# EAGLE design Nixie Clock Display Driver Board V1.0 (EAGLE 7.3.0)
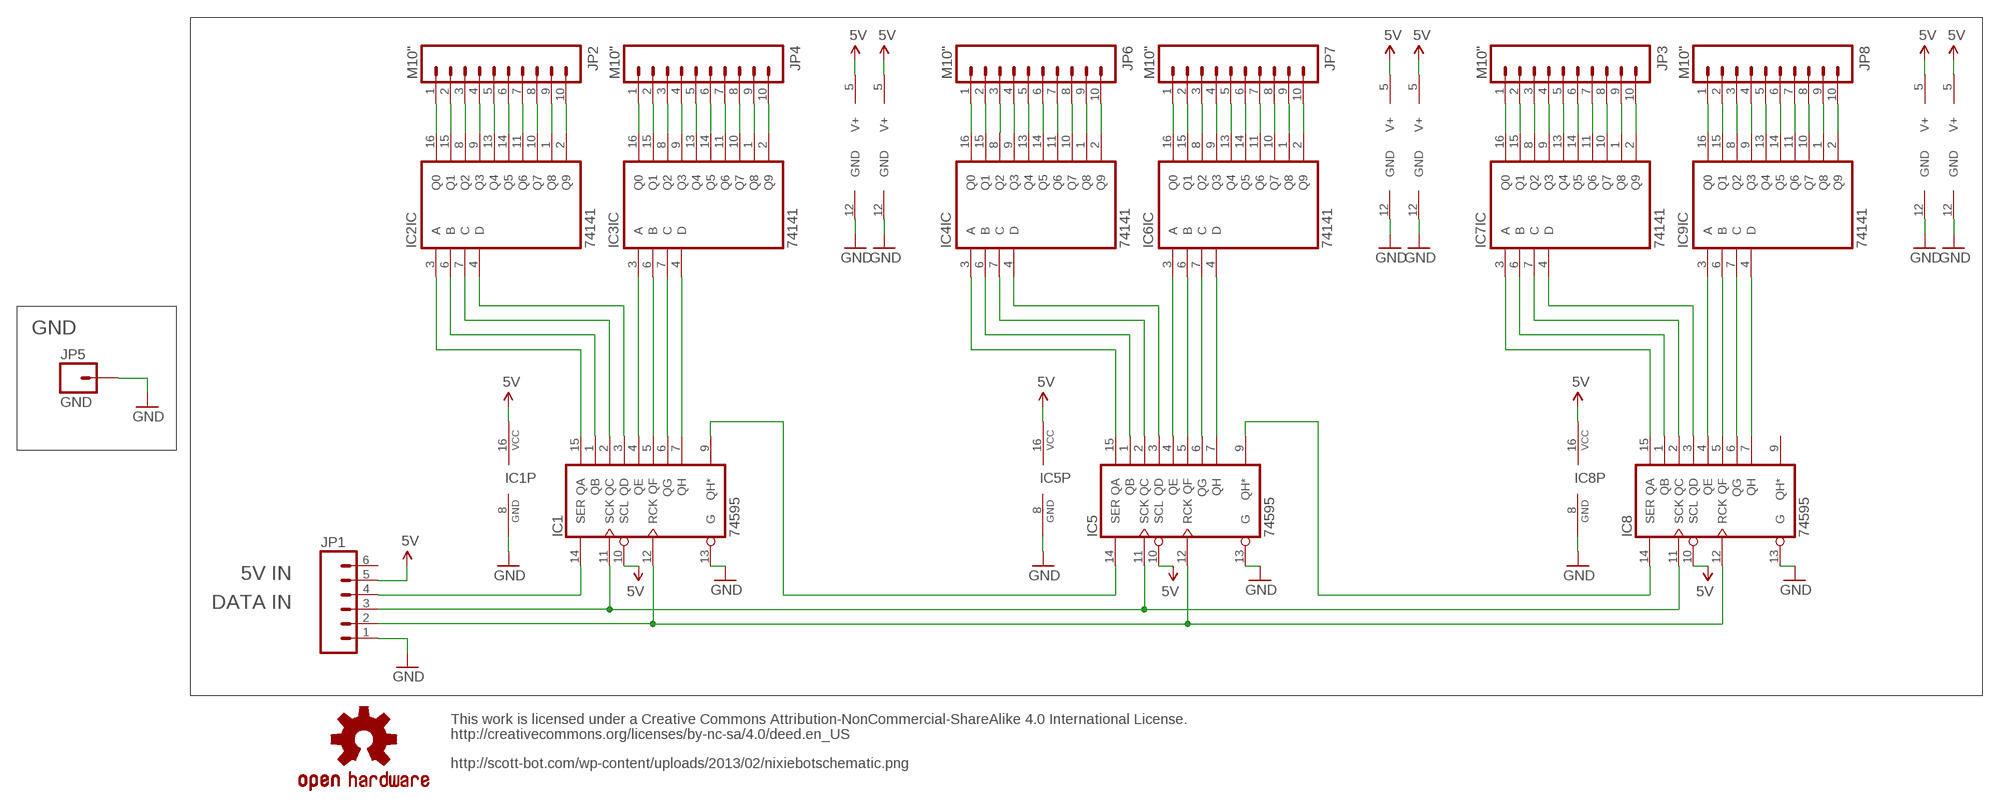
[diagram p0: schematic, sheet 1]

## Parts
IC1  74595  74LS595N  [DIL16]
IC2  74141  IC_74141-DIP-16  [DIL16]
IC3  74141  IC_74141-DIP-16  [DIL16]
IC4  74141  IC_74141-DIP-16  [DIL16]
IC5  74595  74LS595N  [DIL16]
IC6  74141  IC_74141-DIP-16  [DIL16]
IC7  74141  IC_74141-DIP-16  [DIL16]
IC8  74595  74LS595N  [DIL16]
IC9  74141  IC_74141-DIP-16  [DIL16]
JP1  M06NO_SILK  [1X06_NO_SILK]
JP2  M10"  [1X10]
JP3  M10"  [1X10]
JP4  M10"  [1X10]
JP5  GND  M01  [1X01HV]
JP6  M10"  [1X10]
JP7  M10"  [1X10]
JP8  M10"  [1X10]
U$2  OSHW-LOGOM  [OSHW-LOGO-M]

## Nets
5V: IC1.10(SCL) IC1.16(VCC) IC2.5(SUPPLY:V+) IC3.5(SUPPLY:V+) IC4.5(SUPPLY:V+) IC5.10(SCL) IC5.16(VCC) IC6.5(SUPPLY:V+) IC7.5(SUPPLY:V+) IC8.10(SCL) IC8.16(VCC) IC9.5(SUPPLY:V+) JP1.5
GND: IC1.8(GND) IC1.13(G) IC2.12(SUPPLY:GND) IC3.12(SUPPLY:GND) IC4.12(SUPPLY:GND) IC5.8(GND) IC5.13(G) IC6.12(SUPPLY:GND) IC7.12(SUPPLY:GND) IC8.8(GND) IC8.13(G) IC9.12(SUPPLY:GND) JP1.1 JP5.1
IN1: IC1.14(SER) JP1.4
IN2: IC1.12(RCK) IC5.12(RCK) IC8.12(RCK) JP1.2
IN4: IC1.9(QH*) IC5.14(SER)
IN5: IC1.11(SCK) IC5.11(SCK) IC8.11(SCK) JP1.3
IN6: IC5.9(QH*) IC8.14(SER)
N$1: IC2.16(IC:Q0) JP2.1
N$3: IC2.15(IC:Q1) JP2.2
N$4: IC2.8(IC:Q2) JP2.3
N$5: IC2.9(IC:Q3) JP2.4
N$6: IC1.15(QA) IC2.3(IC:A)
N$7: IC2.13(IC:Q4) JP2.5
N$8: IC1.1(QB) IC2.6(IC:B)
N$9: IC1.2(QC) IC2.7(IC:C)
N$10: IC1.3(QD) IC2.4(IC:D)
N$11: IC1.4(QE) IC3.3(IC:A)
N$12: IC2.14(IC:Q5) JP2.6
N$13: IC1.5(QF) IC3.6(IC:B)
N$14: IC1.6(QG) IC3.7(IC:C)
N$15: IC1.7(QH) IC3.4(IC:D)
N$16: IC2.11(IC:Q6) JP2.7
N$17: IC2.10(IC:Q7) JP2.8
N$18: IC2.1(IC:Q8) JP2.9
N$19: IC2.2(IC:Q9) JP2.10
N$20: IC3.16(IC:Q0) JP4.1
N$21: IC3.15(IC:Q1) JP4.2
N$22: IC3.8(IC:Q2) JP4.3
N$23: IC3.9(IC:Q3) JP4.4
N$24: IC3.13(IC:Q4) JP4.5
N$25: IC3.14(IC:Q5) JP4.6
N$26: IC3.11(IC:Q6) JP4.7
N$27: IC3.10(IC:Q7) JP4.8
N$28: IC3.1(IC:Q8) JP4.9
N$29: IC3.2(IC:Q9) JP4.10
N$31: IC4.3(IC:A) IC5.15(QA)
N$32: IC4.6(IC:B) IC5.1(QB)
N$33: IC4.7(IC:C) IC5.2(QC)
N$34: IC4.4(IC:D) IC5.3(QD)
N$35: IC5.4(QE) IC6.3(IC:A)
N$36: IC5.5(QF) IC6.6(IC:B)
N$37: IC5.6(QG) IC6.7(IC:C)
N$38: IC5.7(QH) IC6.4(IC:D)
N$39: IC4.16(IC:Q0) JP6.1
N$40: IC4.15(IC:Q1) JP6.2
N$41: IC4.8(IC:Q2) JP6.3
N$42: IC4.9(IC:Q3) JP6.4
N$43: IC4.13(IC:Q4) JP6.5
N$44: IC4.14(IC:Q5) JP6.6
N$45: IC4.11(IC:Q6) JP6.7
N$46: IC4.10(IC:Q7) JP6.8
N$47: IC4.1(IC:Q8) JP6.9
N$48: IC4.2(IC:Q9) JP6.10
N$49: IC6.16(IC:Q0) JP7.1
N$50: IC6.15(IC:Q1) JP7.2
N$51: IC6.8(IC:Q2) JP7.3
N$52: IC6.9(IC:Q3) JP7.4
N$53: IC6.13(IC:Q4) JP7.5
N$54: IC6.14(IC:Q5) JP7.6
N$55: IC6.11(IC:Q6) JP7.7
N$56: IC6.10(IC:Q7) JP7.8
N$57: IC6.1(IC:Q8) JP7.9
N$58: IC6.2(IC:Q9) JP7.10
N$59: IC7.3(IC:A) IC8.15(QA)
N$60: IC7.6(IC:B) IC8.1(QB)
N$61: IC7.7(IC:C) IC8.2(QC)
N$62: IC7.4(IC:D) IC8.3(QD)
N$63: IC8.4(QE) IC9.3(IC:A)
N$64: IC8.5(QF) IC9.6(IC:B)
N$65: IC8.6(QG) IC9.7(IC:C)
N$66: IC8.7(QH) IC9.4(IC:D)
N$67: IC7.16(IC:Q0) JP3.1
N$68: IC7.15(IC:Q1) JP3.2
N$69: IC7.8(IC:Q2) JP3.3
N$70: IC7.9(IC:Q3) JP3.4
N$71: IC7.13(IC:Q4) JP3.5
N$72: IC7.14(IC:Q5) JP3.6
N$73: IC7.11(IC:Q6) JP3.7
N$74: IC7.10(IC:Q7) JP3.8
N$75: IC7.1(IC:Q8) JP3.9
N$76: IC7.2(IC:Q9) JP3.10
N$77: IC9.16(IC:Q0) JP8.1
N$78: IC9.15(IC:Q1) JP8.2
N$79: IC9.8(IC:Q2) JP8.3
N$80: IC9.9(IC:Q3) JP8.4
N$81: IC9.13(IC:Q4) JP8.5
N$82: IC9.14(IC:Q5) JP8.6
N$83: IC9.11(IC:Q6) JP8.7
N$84: IC9.10(IC:Q7) JP8.8
N$85: IC9.1(IC:Q8) JP8.9
N$86: IC9.2(IC:Q9) JP8.10
Unconnected: IC8.9(QH*) JP1.6

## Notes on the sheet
- GND
- 5V IN
- DATA IN
- This work is licensed under a Creative Commons Attribution-NonCommercial-ShareAlike 4.0 International License.
  http://creativecommons.org/licenses/by-nc-sa/4.0/deed.en_US
- http://scott-bot.com/wp-content/uploads/2013/02/nixiebotschematic.png

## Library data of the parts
IC1 IC5 IC8 = 74xx-us:74*595: 8-bit SHIFT REGISTER, output latch
IC2-IC4 IC6 IC7 IC9 = dp_devices:IC_74141: BCD to decimal decoder
JP1 = SparkFun-Connectors:M06: Header 6 Standard 6-pin 0.1" header. Use with straight break away headers (SKU : PRT-00116), right angle break away headers (PRT-00553), swiss pins (PRT-00743), machine pins (PRT-00117), and female headers (PRT-00115). Molex polarized connector foot print use with SKU : PRT-08094 with associated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
JP2-JP4 JP6-JP8 = SparkFun-Connectors:M10: Header 10 Standard 10-pin 0.1" header. Use with straight break away headers (SKU : PRT-00116), right angle break away headers (PRT-00553), swiss pins (PRT-00743), machine pins (PRT-00117), and female headers (PRT-00115).
JP5 = SparkFun-Connectors:M01: Header 1
U$2 = SparkFun:OSHW-LOGO: Open Source Hardware Logo This logo indicates the piece of hardware it is found on incorporates a OSHW license and/or adheres to the definition of open source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

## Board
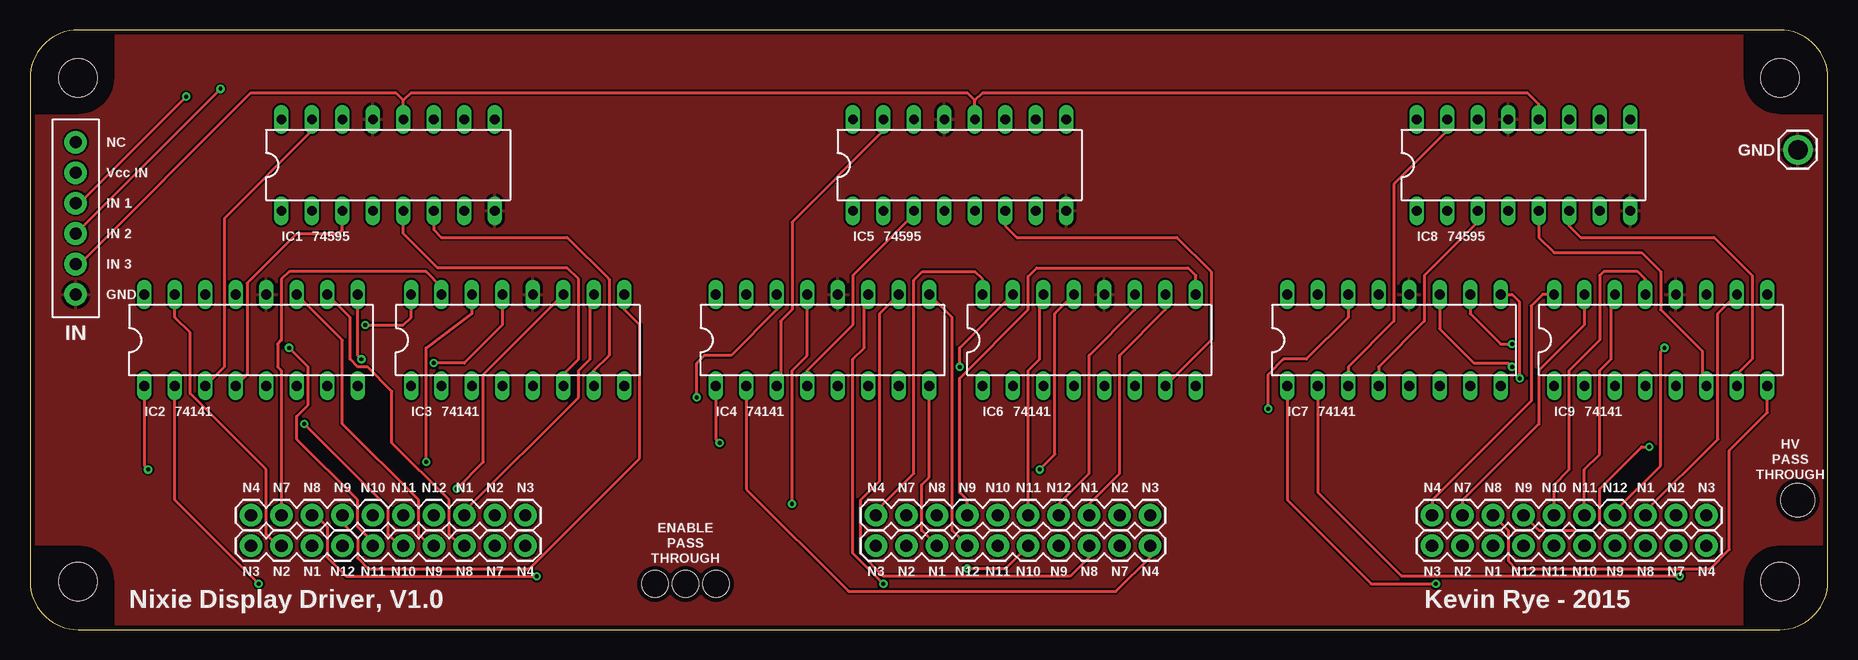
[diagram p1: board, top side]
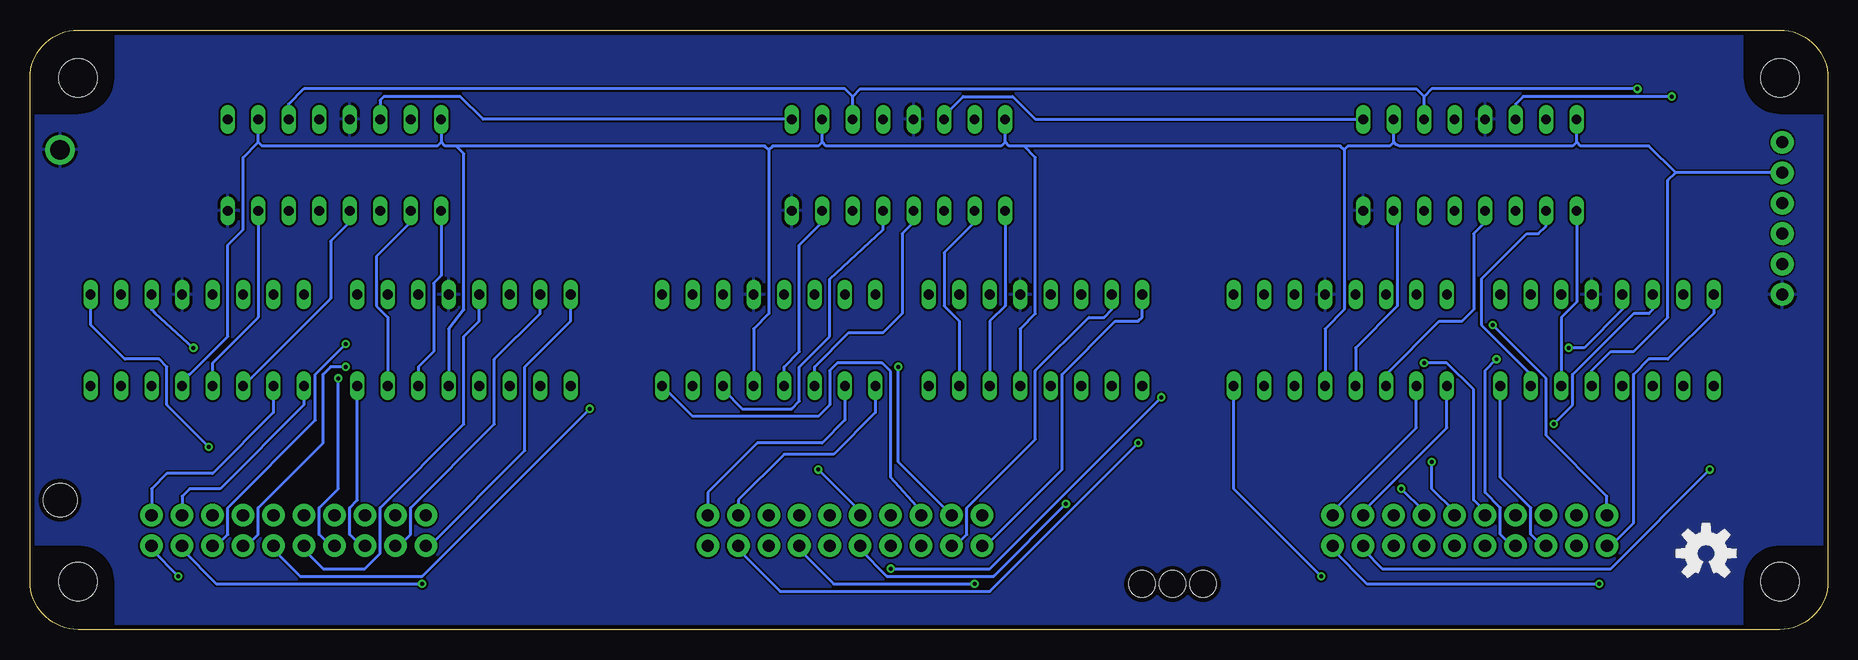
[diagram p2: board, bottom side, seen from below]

Size 149.83 x 50 mm. Coordinates in mm from the lower left corner, seen from the top.
Copper layers (1*16): Top 0.0356mm / dielectric 1.5011mm / Bottom 0.0356mm
Design rules "LaenPCBOrder *": minimum track width 10mil, minimum drill 13mil, track to track 6mil, track to pad 6mil, pad to pad 6mil, via to via 6mil, smd to smd 6mil, copper to edge 15mil, drill to drill 6mil, minimum pad ring 7mil, minimum via ring 7mil, stop-mask expansion 3mil, vias tented up to drill 0mil, thermal gap 10mil
Holes 2.8 mm at 147.32,10.79
Holes 2.2 mm at 52.07,3.81 54.61,3.81 57.15,3.81

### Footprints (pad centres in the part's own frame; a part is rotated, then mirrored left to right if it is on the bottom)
DIL16 = drill 0.813 long: 1 -8.89,-3.81; 2 -6.35,-3.81; 3 -3.81,-3.81; 4 -1.27,-3.81; 5 1.27,-3.81; 6 3.81,-3.81; 7 6.35,-3.81; 8 8.89,-3.81; 9 8.89,3.81; 10 6.35,3.81; 11 3.81,3.81; 12 1.27,3.81; 13 -1.27,3.81; 14 -3.81,3.81; 15 -6.35,3.81; 16 -8.89,3.81
1X06_NO_SILK = drill 1.016 pad 1.88: 1 0,0; 2 2.54,0; 3 5.08,0; 4 7.62,0; 5 10.16,0; 6 12.7,0
1X10 = drill 1.016 pad 1.88: 1 0,0; 2 2.54,0; 3 5.08,0; 4 7.62,0; 5 10.16,0; 6 12.7,0; 7 15.24,0; 8 17.78,0; 9 20.32,0; 10 22.86,0
1X01HV = drill 1.628 pad 2.464: 1 0,0
50X150 = hole 3.2: 4,4; 145.83,4; 145.83,46; 4,46

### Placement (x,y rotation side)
IC1  29.84,38.73 0 top
IC2  18.41,24.13 0 top
IC3  40.64,24.13 0 top
IC4  66.04,24.13 0 top
IC5  77.47,38.73 0 top
IC6  88.27,24.13 0 top
IC7  113.67,24.13 0 top
IC8  124.46,38.73 0 top
IC9  135.89,24.13 0 top
JP1  3.81,27.94 90 top
JP2  18.41,6.99 0 top
JP3  116.84,6.99 0 top
JP4  18.41,9.53 0 top
JP5  147.32,40.01 0 top
JP6  70.48,6.99 0 top
JP7  70.48,9.53 0 top
JP8  116.84,9.53 0 top
U$2  10.16,6.35 0 bottom
U$5  [50X150]  0,0 0 top

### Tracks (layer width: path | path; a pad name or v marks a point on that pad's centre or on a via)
5V
  Bottom 0.254: IC7.5 114.94,25.08 113.67,26.67 113.67,39.69 114.3,40.32 | IC9.5 137.16,21.27 136.53,21.27 133.35,24.45 133.35,32.07 132.08,33.34 132.08,39.37 130.81,40.64 | IC4.5 67.31,25.08 66.04,26.35 66.04,39.37 66.99,40.32 | 68.58,41.59 IC5.16 68.58,40.64 | IC6.5 89.53,25.08 88.27,26.35 88.27,40.01 | IC3.5 41.91,25.08 40.32,26.67 40.32,40.01 | 36.2,40.64 36.01,40.45 35.69,40.32 21.27,40.32 20.95,40.64 | 36.2,40.64 IC1.10 | JP1.5 12.7,38.1 | 130.81,40.64 IC8.10 | IC8.16 115.57,40.64 | 36.2,40.64 36.51,40.32 40.01,40.32 40.32,40.01 | 40.32,40.01 40.64,40.32 66.99,40.32 | 66.99,40.32 68.26,40.32 68.58,40.64 | 68.58,40.64 68.9,40.32 83.5,40.32 83.82,40.64 | 83.82,40.64 IC5.10 | 83.82,40.64 84.14,40.32 87.95,40.32 88.27,40.01 | 88.27,40.01 88.58,40.32 114.3,40.32 | 114.3,40.32 115.25,40.32 115.57,40.64 | 115.57,40.64 115.89,40.32 130.49,40.32 130.81,40.64 | 12.7,38.1 14.92,40.32 20.64,40.32 20.95,40.64 | 20.95,40.64 IC1.16 | IC2.5 19.68,21.59 18.1,23.18 16.19,23.18 13.34,26.04 13.34,37.47 12.7,38.1
GND
  pour Top: -1.27,51.44 151.13,51.44 151.13,-1.27 -1.27,-1.27
  pour Bottom: -0.64,50.8 150.5,50.8 150.5,-0.64 -0.64,-0.64
IN1  (via drill 0.33)
  Top 0.254: v13.02,44.45 4.13,35.56 JP1.4
  Bottom 0.254: v13.02,44.45 25.4,44.45 26.04,43.81 IC1.14
IN2
  Top 0.254: JP1.2 4.13,30.48 18.41,44.77 30.48,44.77 31.11,44.13 | IC1.12 31.11,44.13 | 31.11,44.13 31.75,44.77 78.11,44.77 78.74,44.13 | IC5.12 78.74,44.13 | 78.74,44.13 79.38,44.77 124.78,44.77 125.73,43.81 IC8.12
IN4
  Bottom 0.254: IC1.9 66.04,42.55 67.94,44.45 72.07,44.45 73.66,42.86 IC5.14
IN5  (via drill 0.33)
  Top 0.254: v15.88,45.09 JP1.3
  Bottom 0.254: 81.28,42.86 IC5.11 81.28,44.45 | IC1.11 33.66,44.45 | IC8.11 128.27,43.81 127,45.09 81.92,45.09 81.28,44.45 | v15.88,45.09 33.02,45.09 33.66,44.45 | 81.28,44.45 80.64,45.09 34.29,45.09 33.66,44.45
IN6
  Bottom 0.254: IC5.9 112.08,42.55 113.98,44.45 120.33,44.45 120.65,44.13 IC8.14
N$1
  Bottom 0.254: JP2.1 18.1,6.99 16.19,8.89 16.19,21.27 14.92,22.54 13.34,22.54 9.53,26.35 IC2.16
N$3
  Top 0.254: JP2.2 20.64,6.99 19.68,7.94 19.68,13.34 13.34,19.68 13.34,24.77 12.06,26.04 IC2.15
N$4
  Bottom 0.254: IC2.8 27.3,12.7 24.77,10.16 24.77,7.94 23.81,6.99 JP2.3
N$5  (via drill 0.33)
  Top 0.254: IC2.9 27.3,22.86 v27.62,22.54
  Bottom 0.254: v27.62,22.54 28.57,21.59 28.57,11.43 27.3,10.16 27.3,7.94 26.35,6.99 JP2.4
N$6
  Top 0.254: IC2.3 16.19,21.91 16.19,34.29 23.5,41.59 IC1.15
N$7  (via drill 0.33)
  Top 0.254: v21.59,23.5 23.18,21.91 23.18,18.73 22.23,17.78 22.23,15.88 27.3,10.79 27.3,8.57 28.57,7.3 JP2.5
  Bottom 0.254: IC2.13 17.14,26.67 20.32,23.5 v21.59,23.5
N$8
  Bottom 0.254: IC2.6 22.23,26.04 20.95,27.3 IC1.1
N$9
  Bottom 0.254: IC2.7 24.77,21.27 28.89,25.4 28.89,29.21 25.08,33.02 24.13,33.02 23.5,33.66 IC1.2 23.5,34.61
N$10
  Top 0.254: IC2.4 18.1,21.27 18.1,28.89 22.23,33.02 25.72,33.02 26.04,33.34 IC1.3
N$11
  Bottom 0.254: IC1.4 28.57,33.97 29.53,33.02 29.53,26.67 30.48,25.72 32.38,25.72 36.83,21.27 IC3.3
N$12  (via drill 0.33)
  Top 0.254: v22.86,17.14 29.84,10.16 29.84,7.94 30.8,6.99 JP2.6
  Bottom 0.254: v22.86,17.14 21.27,18.73 21.27,21.27 16.19,26.35 14.92,26.35 14.61,26.67 IC2.14
N$13
  Top 0.254: IC3.6 44.45,21.27 45.72,22.54 45.72,29.21 44.77,30.16 33.97,30.16 31.11,33.02 IC1.5
N$14
  Top 0.254: IC1.6 33.66,33.34 34.29,32.7 44.77,32.7 48.26,29.21 48.26,22.86 46.99,21.59 IC3.7
N$15
  Bottom 0.254: IC3.4 39.37,23.5 35.88,26.99 35.88,34.61 IC1.7
N$16
  Top 0.254: IC2.11 26.04,24.13 26.04,17.14 32.38,10.79 32.38,7.94 33.34,6.99 JP2.7
N$17
  Top 0.254: IC2.10 26.67,26.04 26.67,22.54 27.3,21.91 28.13,21.91 30.16,19.88 30.16,15.56 34.92,10.79 34.92,7.94 35.88,6.99 JP2.8
N$18  (via drill 0.33)
  Top 0.254: IC2.1 9.53,13.65 v9.84,13.34
  Bottom 0.254: v9.84,13.34 18.1,5.08 37.15,5.08 38.73,6.67 JP2.9
N$19  (via drill 0.33)
  Top 0.254: v19.05,3.81 12.06,10.79 IC2.2
  Bottom 0.254: v19.05,3.81 38.42,3.81 41.27,6.67 JP2.10
N$20  (via drill 0.33)
  Top 0.254: v27.94,25.4 31.11,25.4 31.75,26.04 IC3.16
  Bottom 0.254: v27.94,25.4 23.5,20.95 23.5,16.19 18.41,11.11 JP4.1
N$21
  Top 0.254: IC3.15 34.29,28.57 33.02,29.84 21.59,29.84 20.95,29.21 20.95,24.13 20.64,23.81 20.64,21.91 20.95,21.59 JP4.2
N$22  (via drill 0.33)
  Top 0.254: v42.23,4.45 26.35,4.45 24.77,6.03 24.77,8.57 23.81,9.53 JP4.3
  Bottom 0.254: IC3.8 49.53,11.75 v42.23,4.45
N$23
  Top 0.254: 26.04,9.21 JP4.4 26.04,8.89 27.3,7.62 27.3,5.98 28.2,5.08 41.59,5.08 50.8,14.29 50.8,25.4 49.53,26.67 IC3.9
N$24  (via drill 0.33)
  Top 0.254: IC3.13 39.37,25.4 36.2,22.23 v33.66,22.23
  Bottom 0.254: v33.66,22.23 31.75,22.23 29.53,20 29.53,10.79 28.57,9.84 JP4.5
N$25  (via drill 0.33)
  Top 0.254: v33.02,13.97 33.02,23.5 36.83,26.35 IC3.14
  Bottom 0.254: v33.02,13.97 33.02,11.75 31.11,9.84 JP4.6
N$26  (via drill 0.33)
  Top 0.254: IC3.11 37.78,21.27 37.78,13.97 v35.56,11.75
  Bottom 0.254: v35.56,11.75 33.66,9.84 JP4.7
N$27
  Top 0.254: IC3.10 46.67,27.62 46.67,22.54 45.72,21.59 45.72,19.37 36.2,9.84 JP4.8
N$28
  Bottom 0.254: IC3.1 31.75,16.83 38.73,9.84 JP4.9
N$29
  Bottom 0.254: IC3.2 34.29,16.83 41.27,9.84 JP4.10
N$31
  Top 0.254: IC4.3 62.55,20.64 62.55,25.72 63.5,26.67 63.5,33.97 71.12,41.59 IC5.15
N$32
  Bottom 0.254: IC4.6 69.85,25.72 68.58,26.99 IC5.1
N$33
  Bottom 0.254: IC4.7 72.39,25.72 73.66,26.99 73.66,31.43 71.12,33.97 IC5.2
N$34
  Top 0.254: IC5.3 73.66,34.61 68.58,29.53 68.58,25.4 64.77,21.59 IC4.4
N$35
  Bottom 0.254: IC5.4 76.2,33.97 77.15,33.02 77.15,26.35 78.74,24.77 81.6,24.77 84.45,21.91 IC6.3
N$36
  Bottom 0.254: IC5.5 78.74,33.34 83.19,29.21 83.19,24.45 85.72,21.91 85.72,19.05 86.36,18.41 90.49,18.41 92.08,20 IC6.6
N$37
  Top 0.254: IC6.7 98.42,24.13 98.42,29.84 95.57,32.7 82.23,32.7 81.28,33.66 IC5.6
N$38
  Bottom 0.254: IC5.7 83.82,33.97 85.72,32.07 85.72,23.18 87,21.91 IC6.4
N$39
  Bottom 0.254: JP6.1 70.17,6.99 63.82,13.34 63.82,21.27 59.37,25.72 57.47,25.72 57.15,26.04 IC4.16
N$40
  Bottom 0.254: JP6.2 72.71,6.99 71.75,7.94 71.75,10.16 66.04,15.88 66.04,21.59 61.59,26.04 60.33,26.04 59.69,26.67 IC4.15
N$41
  Top 0.254: JP6.3 74.3,8.26 74.3,12.06 74.93,12.7 IC4.8
N$42
  Top 0.254: IC4.9 76.83,26.04 76.83,8.26 JP6.4
N$43  (via drill 0.33)
  Top 0.254: IC4.13 64.77,22.86 63.5,21.59 v63.5,10.48
  Bottom 0.254: v63.5,10.48 69.53,4.45 78.42,4.45 80.64,6.67 JP6.5
N$44  (via drill 0.33)
  Top 0.254: v55.56,19.37 55.56,22.23 56.2,22.86 58.42,22.86 62.23,26.67 IC4.14 | v78.11,5.08 81.28,5.08 JP6.6
  Bottom 0.254: v55.56,19.37 69.85,5.08 v78.11,5.08
N$45  (via drill 0.33)
  Top 0.254: IC4.11 69.53,27.62 69.53,23.5 68.58,22.54 68.58,6.35 v71.12,3.81
  Bottom 0.254: v71.12,3.81 82.87,3.81 85.72,6.67 JP6.7
N$46
  Top 0.254: IC4.10 70.8,26.35 70.8,12.38 69.22,10.79 69.22,6.35 71.12,4.45 86.68,4.45 88.27,6.03 JP6.8
N$47  (via drill 0.33)
  Top 0.254: IC4.1 57.15,15.88 v57.47,15.56
  Bottom 0.254: v57.47,15.56 69.85,3.17 87.31,3.17 90.81,6.67 JP6.9
N$48
  Top 0.254: IC4.2 59.69,11.71 68.22,3.17 90.49,3.17 93.34,6.03 JP6.10
N$49
  Top 0.254: JP7.1 70.48,9.84 73.66,13.02 73.66,29.14 74.37,29.84 78.74,29.84 79.38,29.21 IC6.16
N$50  (via drill 0.33)
  Top 0.254: IC6.15 77.47,23.5 v77.47,21.91
  Bottom 0.254: JP7.2 77.47,13.97 v77.47,21.91
N$51
  Bottom 0.254: IC6.8 94.61,17.78 84.14,17.78 83.19,18.73 83.19,21.59 82.55,22.23 78.81,22.23 78.11,21.52 78.11,12.7 75.56,9.84 JP7.3
N$52
  Top 0.254: IC6.9 97.16,29.53 96.52,30.16 83.89,30.16 83.19,29.45 83.19,26.67 77.47,20.95 77.47,11.43 78.11,10.79 JP7.4
N$53  (via drill 0.33)
  Top 0.254: IC6.13 85.41,26.35 85.41,14.61 v84.14,13.34
  Bottom 0.254: v84.14,13.34 80.64,9.84 JP7.5
N$54
  Top 0.254: IC6.14 84.14,27.62 84.14,22.54 83.19,21.59 JP7.6
N$55
  Top 0.254: JP7.7 85.72,10.48 88.27,13.02 88.27,22.86 92.08,26.67 IC6.11
N$56
  Top 0.254: JP7.8 88.27,10.48 90.81,13.02 90.81,22.86 94.61,26.67 IC6.10
N$57
  Bottom 0.254: 90.81,9.84 JP7.9 90.81,10.79 87,14.61 82.87,14.61 79.38,18.1 IC6.1
N$58
  Bottom 0.254: 93.34,9.84 JP7.10 93.34,11.43 89.22,15.56 83.82,15.56 81.92,17.46 IC6.2
N$59
  Top 0.254: IC8.15 118.11,41.59 113.67,37.15 113.67,25.72 109.86,21.91 IC7.3
N$60
  Bottom 0.254: IC8.1 115.57,29.53 116.2,28.89 116.2,23.18 117.47,21.91 IC7.6
N$61
  Bottom 0.254: IC7.7 120.02,26.04 120.97,26.99 120.97,31.11 118.11,33.97 IC8.2
N$62
  Top 0.254: IC8.3 120.65,33.97 116.2,29.53 116.2,25.72 112.39,21.91 IC7.4
N$63
  Bottom 0.254: IC9.3 124.78,27.62 124.78,32.38 123.19,33.97 IC8.4
N$64
  Top 0.254: IC9.6 139.38,20.64 139.38,23.18 135.89,26.67 135.89,29.84 134.3,31.43 127,31.43 125.73,32.7 IC8.5
N$65
  Top 0.254: IC9.7 142.24,21.27 143.51,22.54 143.51,29.53 140.34,32.7 129.22,32.7 128.27,33.66 IC8.6
N$66
  Bottom 0.254: IC8.7 130.81,26.04 134.62,22.23 IC9.4
N$67
  Bottom 0.254: JP3.1 116.52,6.99 108.58,14.92 108.58,21.91 104.78,25.72 IC7.16
N$68
  Bottom 0.254: IC7.15 107.31,26.35 111.12,22.54 111.12,17.14 118.11,10.16 118.11,7.94 119.06,6.99 JP3.2
N$69
  Bottom 0.254: IC7.8 122.56,10.79 123.19,10.16 123.19,7.94 122.24,6.99 JP3.3
N$70  (via drill 0.33)
  Top 0.254: v124.14,20.95 124.14,27.3 123.51,27.94 IC7.9
  Bottom 0.254: v124.14,20.95 124.14,11.75 125.73,10.16 125.73,7.94 124.78,6.99 JP3.4
N$71
  Bottom 0.254: JP3.5 127,6.67 125.41,5.08 121.92,5.08 120.65,6.35 120.65,10.16 113.67,17.14 113.67,24.45 112.39,25.72 IC7.13
N$72  (via drill 0.33)
  Top 0.254: v103.19,18.41 103.19,21.27 104.46,22.54 106.36,22.54 109.86,26.04 IC7.14
  Bottom 0.254: v103.19,18.41 117.16,4.45 127.32,4.45 129.54,6.67 JP3.6
N$73  (via drill 0.33)
  Top 0.254: IC7.11 117.47,25.08 120.33,22.23 123.19,22.23 v123.51,21.91
  Bottom 0.254: JP3.7 131.76,6.99 130.81,7.94 130.81,10.16 125.41,15.56 125.41,21.27 124.78,21.91 v123.51,21.91
N$74  (via drill 0.33)
  Top 0.254: IC7.10 120.02,26.35 122.56,23.81 v123.51,23.81
  Bottom 0.254: v123.51,23.81 126.05,21.27 126.05,17.46 133.35,10.16 133.35,7.94 134.3,6.99 JP3.8
N$75  (via drill 0.33)
  Top 0.254: IC7.1 104.78,10.79 111.76,3.81 v117.16,3.81
  Bottom 0.254: v117.16,3.81 134.3,3.81 137.16,6.67 JP3.9
N$76  (via drill 0.33)
  Top 0.254: v137.48,4.45 114.3,4.45 107.31,11.43 IC7.2
  Bottom 0.254: v137.48,4.45 139.7,6.67 JP3.10
N$77
  Top 0.254: IC9.16 126.05,27.94 125.09,26.99 125.09,19.05 116.84,10.79 JP8.1
N$78
  Top 0.254: JP8.2 119.38,10.79 125.73,17.14 125.73,21.59 129.54,25.4 IC9.15
N$79
  Top 0.254: JP8.3 123.19,8.26 123.19,5.71 123.83,5.08 140.02,5.08 141.6,6.67 141.6,14.92 144.78,18.1 IC9.8
N$80  (via drill 0.33)
  Top 0.254: JP8.4 125.73,8.26 130.18,8.26 130.81,8.89 130.81,11.75 134.3,15.24 v134.94,15.24
  Bottom 0.254: v134.94,15.24 138.43,18.73 138.43,21.91 139.06,22.54 141.92,22.54 144.78,25.4 IC9.9
N$81
  Top 0.254: JP8.5 127,12.06 128.27,13.34 128.27,21.59 130.81,24.13 130.81,29.53 131.13,29.84 133.99,29.84 134.62,29.21 IC9.13
N$82
  Top 0.254: IC9.14 131.76,27.62 131.76,22.54 130.81,21.59 130.81,14.61 129.54,13.34 JP8.6
N$83  (via drill 0.33)
  Top 0.254: v136.21,23.5 135.89,23.18 135.89,13.65 132.08,9.84 JP8.7
  Bottom 0.254: IC9.11 139.7,26.67 139.38,26.35 v136.21,23.5
N$84
  Top 0.254: IC9.10 140.65,26.35 140.65,15.88 134.62,9.84 JP8.8
N$85
  Bottom 0.254: 137.16,9.84 JP8.9 137.16,11.11 136.53,11.75 133.99,11.75 127,18.73 IC9.1
N$86
  Bottom 0.254: 139.7,9.84 JP8.10 139.7,11.75 138.43,13.02 134.62,13.02 129.54,18.1 IC9.2

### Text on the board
Unrouted: This work is licensed under a Creative Commons Attribution-NonCommercial-ShareAlike 4.0 International License. / http://creativecommons.org/licenses/by-nc-sa/4.0/deed.en_US
tNames: NC | Vcc IN | IN 1 | IN 2 | IN 3 | GND | IN | HV | PASS | THROUGH | N4 | N7 | N8 | N9 | N10 | N11 | N12 | N1 | N2 | N3 | N4 | N7 | N8 | N9 | N10 | N11 | N12 | N1 | N2 | N3 | N4 | N7 | N8 | N9 | N10 | N11 | N12 | N1 | N2 | N3 | ENABLE | PASS | THROUGH | N3 | N2 | N1 | N12 | N11 | N10 | N9 | N8 | N7 | N4 | N3 | N2 | N1 | N12 | N11 | N10 | N9 | N8 | N7 | N4 | N3 | N2 | N1 | N12 | N11 | N10 | N9 | N8 | N7 | N4 | Nixie Display Driver, V1.0 | Kevin Rye - 2015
